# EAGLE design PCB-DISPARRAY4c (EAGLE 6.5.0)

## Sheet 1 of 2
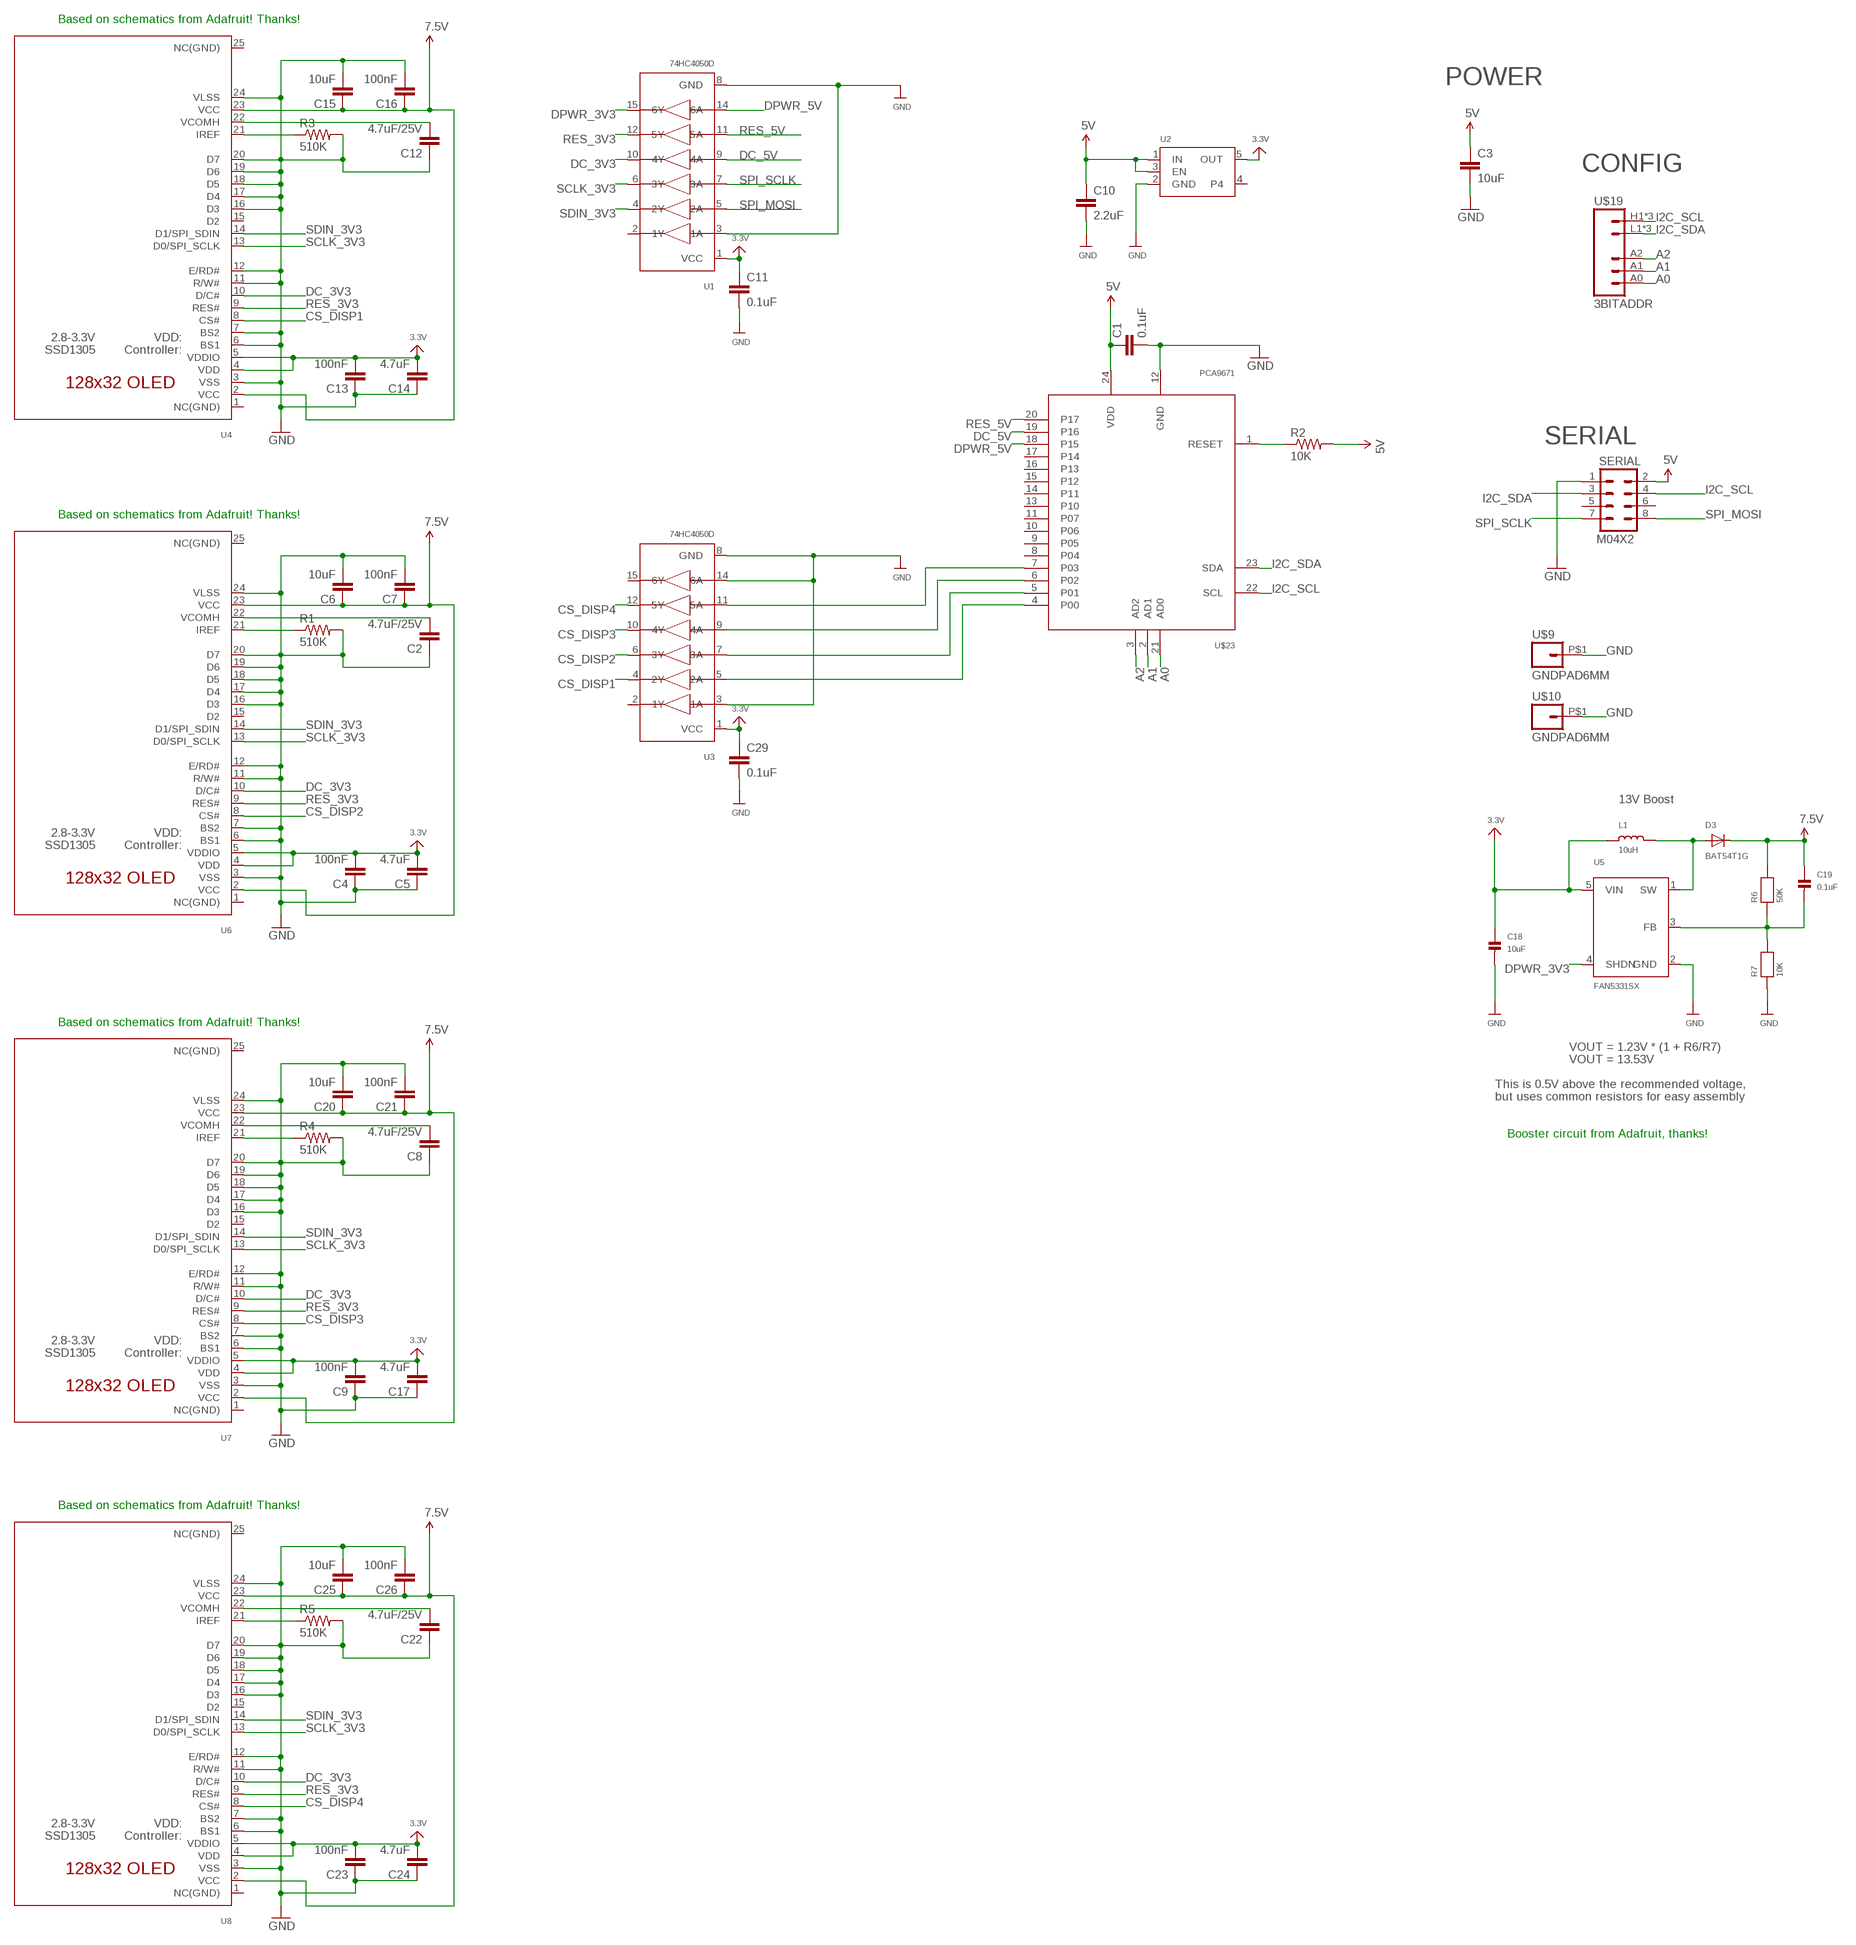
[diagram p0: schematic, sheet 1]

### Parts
C1  0.1uF  CAP0603-CAP  [0603-CAP]
C2  4.7uF/25V  CAP0805  [0805]
C3  10uF  CAP0805  [0805]
C4  100nF  CAP0603-CAP  [0603-CAP]
C5  4.7uF  CAP0603-CAP  [0603-CAP]
C6  10uF  CAP0805  [0805]
C7  100nF  CAP0805  [0805]
C8  4.7uF/25V  CAP0805  [0805]
C9  100nF  CAP0603-CAP  [0603-CAP]
C10  2.2uF  CAP0603-CAP  [0603-CAP]
C11  0.1uF  CAP0603-CAP  [0603-CAP]
C12  4.7uF/25V  CAP0805  [0805]
C13  100nF  CAP0603-CAP  [0603-CAP]
C14  4.7uF  CAP0603-CAP  [0603-CAP]
C15  10uF  CAP0805  [0805]
C16  100nF  CAP0603-CAP  [0603-CAP]
C17  4.7uF  CAP0603-CAP  [0603-CAP]
C18  10uF  CAP_CERAMIC0805  [0805]
C19  0.1uF  CAP_CERAMIC0603  [0603]
C20  10uF  CAP0805  [0805]
C21  100nF  CAP0603-CAP  [0603-CAP]
C22  4.7uF/25V  CAP0805  [0805]
C23  100nF  CAP0603-CAP  [0603-CAP]
C24  4.7uF  CAP0603-CAP  [0603-CAP]
C25  10uF  CAP0805  [0805]
C26  100nF  CAP0603-CAP  [0603-CAP]
C29  0.1uF  CAP0603-CAP  [0603-CAP]
D3  BAT54T1G  DIODESOD-123  [SOD-123]
L1  10uH  INDUCTOR  [INDUCTOR_1007]
R1  510K  RESISTOR0603-RES  [0603-RES]
R2  10K  RESISTOR0603-RES  [0603-RES]
R3  510K  RESISTOR0603-RES  [0603-RES]
R4  510K  RESISTOR0603-RES  [0603-RES]
R5  510K  RESISTOR0603-RES  [0603-RES]
R6  50K  RESISTOR0603  [0603]
R7  10K  RESISTOR0603  [0603]
SERIAL  M04X2  [2X4]
U1  74HC4050D  74HC4050DTSSOP16  [TSSOP16]
U2  VREG_SOT23-5  [SOT23-5]
U3  74HC4050D  74HC4050DTSSOP16  [TSSOP16]
U4  ER-OLED0.91-2TOP  [ER_OLED0.91-2]
U5  FAN5331SX  FAN5331  [SOT23-5]
U6  ER-OLED0.91-2TOP  [ER_OLED0.91-2]
U7  ER-OLED0.91-2TOP  [ER_OLED0.91-2]
U8  ER-OLED0.91-2TOP  [ER_OLED0.91-2]
U$9  GNDPAD6MM  [3.2MMPAD6MM]
U$10  GNDPAD6MM  [3.2MMPAD6MM]
U$19  3BITADDR  [3BITADDR]
U$23  PCA9671  [TSSOP24]

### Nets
3.3V [Power]: C4.2 C5.2 C9.2 C11.1 C13.2 C14.2 C17.2 C18.1 C23.2 C24.2 C29.1 L1.P$1 U1.1(VCC) U2.5(OUT) U3.1(VCC) U4.4(VDD) U4.5(VDDIO) U5.5(VIN) U6.4(VDD) U6.5(VDDIO) U7.4(VDD) U7.5(VDDIO) U8.4(VDD) U8.5(VDDIO)
5V [Power]: C1.1 C3.1 C10.1 R2.2 SERIAL.2 U2.1(IN) U2.3(EN) U$23.24(VDD)
7.5V [Power]: C6.1 C7.1 C15.1 C16.1 C19.1 C20.1 C21.1 C25.1 C26.1 D3.C R6.2 U4.2(VCC) U4.23(VCC) U6.2(VCC) U6.23(VCC) U7.2(VCC) U7.23(VCC) U8.2(VCC) U8.23(VCC)
A0: U$19.A0 U$23.21(AD0)
A1: U$19.A1 U$23.2(AD1)
A2: U$19.A2 U$23.3(AD2)
CS_DISP1: U3.4(2Y) U4.8(CS#)
CS_DISP2: U3.6(3Y) U6.8(CS#)
CS_DISP3: U3.10(4Y) U7.8(CS#)
CS_DISP4: U3.12(5Y) U8.8(CS#)
DC_3V3: U1.10(4Y) U4.10(D/C#) U6.10(D/C#) U7.10(D/C#) U8.10(D/C#)
DC_5V: U1.9(4A) U$23.19(P16)
DPWR_3V3: U1.15(6Y) U5.4(SHDN)
DPWR_5V: U1.14(6A) U$23.18(P15)
GND [Power]: C1.2 C2.1 C3.2 C4.1 C5.1 C6.2 C7.2 C8.1 C9.1 C10.2 C11.2 C12.1 C13.1 C14.1 C15.2 C16.2 C17.1 C18.2 C20.2 C21.2 C22.1 C23.1 C24.1 C25.2 C26.2 C29.2 R1.2 R3.2 R4.2 R5.2 R7.1 SERIAL.1 U1.3(1A) U1.8(GND) U2.2(GND) U3.3(1A) U3.8(GND) U3.14(6A) U4.3(VSS) U4.6(BS1) U4.7(BS2) U4.11(R/W#) U4.12(E/RD#) U4.16(D3) U4.17(D4) U4.18(D5) U4.19(D6) U4.20(D7) U4.24(VLSS) U5.2(GND) U6.3(VSS) U6.6(BS1) U6.7(BS2) U6.11(R/W#) U6.12(E/RD#) U6.16(D3) U6.17(D4) U6.18(D5) U6.19(D6) U6.20(D7) U6.24(VLSS) U7.3(VSS) U7.6(BS1) U7.7(BS2) U7.11(R/W#) U7.12(E/RD#) U7.16(D3) U7.17(D4) U7.18(D5) U7.19(D6) U7.20(D7) U7.24(VLSS) U8.3(VSS) U8.6(BS1) U8.7(BS2) U8.11(R/W#) U8.12(E/RD#) U8.16(D3) U8.17(D4) U8.18(D5) U8.19(D6) U8.20(D7) U8.24(VLSS) U$9.P$1 U$10.P$1 U$23.12(GND)
I2C_SCL: SERIAL.4 U$19.H1(VCC) U$19.H2(VCC) U$19.H3(VCC) U$23.22(SCL)
I2C_SDA: SERIAL.3 U$19.L1(GND) U$19.L2(GND) U$19.L3(GND) U$23.23(SDA)
N$1: R2.1 U$23.1(RESET)
N$2: R1.1 U6.21(IREF)
N$3: C2.2 U6.22(VCOMH)
N$4: R4.1 U7.21(IREF)
N$5: R3.1 U4.21(IREF)
N$6: C8.2 U7.22(VCOMH)
N$7: R5.1 U8.21(IREF)
N$8: C22.2 U8.22(VCOMH)
N$10: C12.2 U4.22(VCOMH)
N$14 [Power]: D3.A L1.P$2 U5.1(SW)
N$15: C19.2 R6.1 R7.2 U5.3(FB)
N$29: U3.5(2A) U$23.4(P00)
N$30: U3.7(3A) U$23.5(P01)
N$31: U3.9(4A) U$23.6(P02)
N$32: U3.11(5A) U$23.7(P03)
RES_3V3: U1.12(5Y) U4.9(RES#) U6.9(RES#) U7.9(RES#) U8.9(RES#)
RES_5V: U1.11(5A) U$23.20(P17)
SCLK_3V3: U1.6(3Y) U4.13(D0/SPI_SCLK) U6.13(D0/SPI_SCLK) U7.13(D0/SPI_SCLK) U8.13(D0/SPI_SCLK)
SDIN_3V3: U1.4(2Y) U4.14(D1/SPI_SDIN) U6.14(D1/SPI_SDIN) U7.14(D1/SPI_SDIN) U8.14(D1/SPI_SDIN)
SPI_MOSI: SERIAL.8 U1.5(2A)
SPI_SCLK: SERIAL.7 U1.7(3A)
Unconnected: SERIAL.5 SERIAL.6 U1.2(1Y) U2.4 U3.2(1Y) U3.15(6Y) U4.1(NC(GND)) U4.15(D2) U4.25(NC(GND)) U6.1(NC(GND)) U6.15(D2) U6.25(NC(GND)) U7.1(NC(GND)) U7.15(D2) U7.25(NC(GND)) U8.1(NC(GND)) U8.15(D2) U8.25(NC(GND)) U$23.8(P04) U$23.9(P05) U$23.10(P06) U$23.11(P07) U$23.13(P10) U$23.14(P11) U$23.15(P12) U$23.16(P13) U$23.17(P14)

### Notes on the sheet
- Based on schematics from Adafruit! Thanks!
- POWER
- CONFIG
- SERIAL
- Based on schematics from Adafruit! Thanks!
- 13V Boost
- Based on schematics from Adafruit! Thanks!
- VOUT = 1.23V * (1 + R6/R7)
- VOUT = 13.53V
- This is 0.5V above the recommended voltage,
- but uses common resistors for easy assembly
- Booster circuit from Adafruit, thanks!
- Based on schematics from Adafruit! Thanks!

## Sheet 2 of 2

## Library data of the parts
C1-C17 C20-C26 C29 = SparkFun:CAP: Capacitor
C18 C19 = microbuilder:CAP_CERAMIC: Ceramic Capacitors
D3 = microbuilder:DIODE: Diode
L1 = microbuilder:INDUCTOR: Inductors
R1-R5 = SparkFun:RESISTOR: Resistor
R6 R7 = microbuilder:RESISTOR: Resistors
SERIAL = SparkFun:M04X2
U1 U3 = SKAARHOJ:74HC4050D: 6-channel level shifter 74HC4050D - 2V-6V Supply Digikey: 74HC4050D,653-ND Mouser: 771-74HC4050D-T
U2 = microbuilder:VREG_SOT23-5: SOT23-5 Fixed Voltage Regulators To better organise some of the SOT23-5 fixed voltage regulators in this library, this new part was created. Part Current Out V Out V In V Dropout Digikey Part No. ADP121 150mA 3.3V 3.4-5.5V 0.09V @ 150mA ADP121-AUJZ33R7CT-ND ADP121 150mA 3.0V 3.1-5.5V 0.09V @ 150mA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
U4 U6-U8 = SKAARHOJ:ER-OLED0.91-2: UG-2864HSWEG01 OLED display Both 1.3" and 0.96" models share the same FPC tab footprint, only the screen dimensions vary.
U5 = microbuilder:FAN5331: FAN5331 - LED/OLED 20V Boost Converter Digikey: FAN5331SXCT-ND
U$9 U$10 = SKAARHOJ:GNDPAD
U$19 = SKAARHOJ:3BITADDR
U$23 = SKAARHOJ:PCA9671

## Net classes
0 default: width 0.203 mm, drill 0.305 mm, clearance 0.152 mm
1 Power: width 0.305 mm, drill 0.406 mm, clearance 0.152 mm

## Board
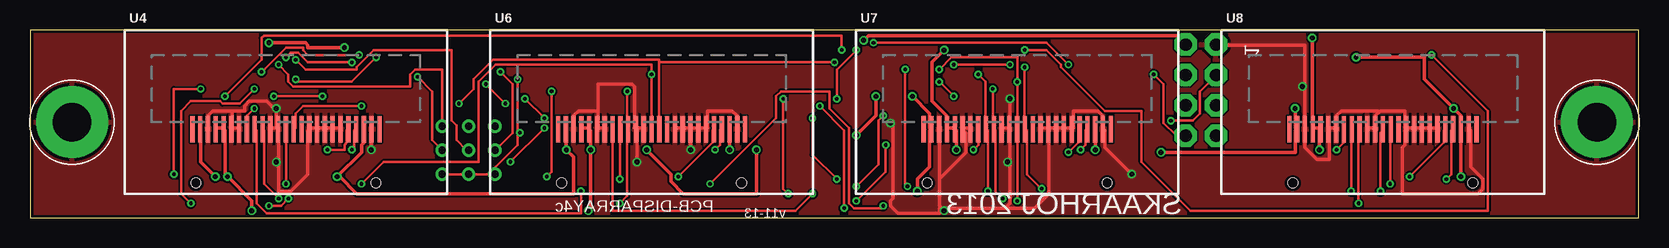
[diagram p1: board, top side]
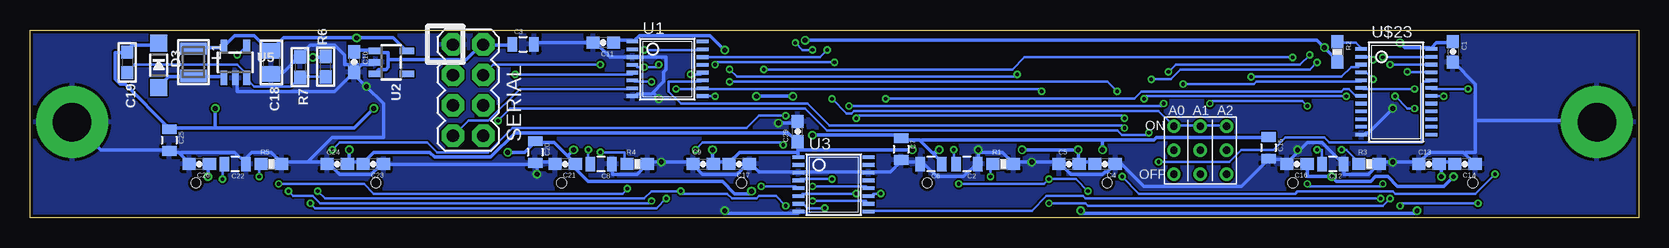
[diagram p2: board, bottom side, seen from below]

Size 134.11 x 15.7 mm. Coordinates in mm from the lower left corner, seen from the top.
Outline: 134.11,0 134.11,15.7 0,15.7 0,0 134.11,0
Copper layers (1*16): Top 0.035mm / dielectric 1.5mm / Bottom 0.035mm
Design rules "Fusion_eagle_rule_v1.1": minimum track width 6mil, minimum drill 12mil, track to track 6mil, track to pad 6mil, pad to pad 6mil, via to via 6mil, smd to smd 0mil, copper to edge 10mil, drill to drill 10mil, minimum pad ring 10mil, minimum via ring 6mil, stop-mask expansion 2mil, vias tented up to drill 100mil, thermal gap 10mil

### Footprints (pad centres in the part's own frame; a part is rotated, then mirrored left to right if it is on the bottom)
0603-CAP = smd 1.1 x 1: 1 -0.85,0; 2 0.85,0
0805 = smd 0.8 x 1.2: 1 -0.9,0; 2 0.9,0
0805' = smd 1.3 x 1.5: 1 -0.95,0; 2 0.95,0
0603 = smd 1.1 x 1: 1 -0.85,0; 2 0.85,0
SOD-123 = smd 1.4 x 1.4: A 1.85,0; C -1.85,0
INDUCTOR_1007 = smd 1.016 x 2.2: P$1 -1.127,0; P$2 1.127,0
0603-RES = smd 1.1 x 1: 1 -0.85,0; 2 0.85,0
2X4 = drill 1.016 pad 1.88 octagon: 1 -3.81,-1.27; 2 -3.81,1.27; 3 -1.27,-1.27; 4 -1.27,1.27; 5 1.27,-1.27; 6 1.27,1.27; 7 3.81,-1.27; 8 3.81,1.27
TSSOP16 = smd 0.305 x 0.991: 1 -3.575,-2.918; 2 -2.925,-2.918; 3 -2.275,-2.918; 4 -1.625,-2.918; 5 -0.975,-2.918; 6 -0.325,-2.918; 7 0.325,-2.918; 8 0.975,-2.918; 9 0.975,2.918; 10 0.325,2.918; 11 -0.325,2.918; 12 -0.975,2.918; 13 -1.625,2.918; 14 -2.275,2.918; 15 -2.925,2.918; 16 -3.575,2.918
SOT23-5 = smd 0.55 x 1.2: 1 -0.95,-1.3; 2 0,-1.3; 3 0.95,-1.3; 4 0.95,1.3; 5 -0.95,1.3
ER_OLED0.91-2 = smd 0.35 x 2.2: 1 -7.8,-1.43; 2 -7.15,-1.43; 3 -6.5,-1.43; 4 -5.85,-1.43; 5 -5.2,-1.43; 6 -4.55,-1.43; 7 -3.9,-1.43; 8 -3.25,-1.43; 9 -2.6,-1.43; 10 -1.95,-1.43; 11 -1.3,-1.43; 12 -0.65,-1.43; 13 0,-1.43; 14 0.65,-1.43; 15 1.3,-1.43; 16 1.95,-1.43; 17 2.6,-1.43; 18 3.25,-1.43; 19 3.9,-1.43; 20 4.55,-1.43; 21 5.2,-1.43; 22 5.85,-1.43; 23 6.5,-1.43; 24 7.15,-1.43; 25 7.8,-1.43 | hole 0.8: -7.5,-5.93; 7.5,-5.93
3.2MMPAD6MM = drill 3.2 pad 6: P$1 0,0
3BITADDR = drill 0.6: A0 -2.2,0; A1 0,0; A2 2.2,0; H1 -2.2,2; H2 0,2; H3 2.2,2; L1 -2.2,-2; L2 0,-2; L3 2.2,-2
TSSOP24 = smd 0.305 x 0.991: 1 -4.225,-2.918; 2 -3.575,-2.918; 3 -2.925,-2.918; 4 -2.275,-2.918; 5 -1.625,-2.918; 6 -0.975,-2.918; 7 -0.325,-2.918; 8 0.325,-2.918; 9 0.975,-2.918; 10 1.625,-2.918; 11 2.275,-2.918; 12 2.925,-2.918; 13 2.925,2.918; 14 2.275,2.918; 15 1.625,2.918; 16 0.975,2.918; 17 0.325,2.918; 18 -0.325,2.918; 19 -0.975,2.918; 20 -1.625,2.918; 21 -2.275,2.918; 22 -2.925,2.918; 23 -3.575,2.918; 24 -4.225,2.918

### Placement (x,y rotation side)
C1  15.49,13.87 270 bottom
C2  56,4.5 180 bottom
C3  93,14.5 0 bottom
C4  44.5,4.5 180 bottom
C5  47.5,4.5 0 bottom
C6  59,4.5 180 bottom
C7  61.5,5.75 270 bottom
C8  86.5,4.5 180 bottom
C9  78,4.5 0 bottom
C10  107.09,13.02 270 bottom
C11  86.32,14.63 180 bottom
C12  25.5,4.5 180 bottom
C13  17.5,4.5 0 bottom
C14  14.5,4.5 180 bottom
C15  30.87,5.87 270 bottom
C16  28.5,4.5 180 bottom
C17  75,4.5 180 bottom
C18  10uF  [0805']  114,13 270 bottom
C19  126,13 270 bottom
C20  92,5.5 270 bottom
C21  89.5,4.5 180 bottom
C22  117,4.5 180 bottom
C23  105.5,4.5 180 bottom
C24  108.5,4.5 0 bottom
C25  122.5,6.5 270 bottom
C26  120,4.5 180 bottom
C29  70.12,7.21 90 bottom
D3  123.37,12.75 270 bottom
L1  120.5,13 270 bottom
R1  53,4.5 0 bottom
R2  25.13,13.88 270 bottom
R3  22.5,4.5 0 bottom
R4  83.5,4.5 0 bottom
R5  114,4.5 0 bottom
R6  109.46,12.64 90 bottom
R7  111.61,12.59 270 bottom
SERIAL  97.6,10.67 270 bottom
U1  80.98,11.16 270 bottom
U2  104,13 270 bottom
U3  67.12,1.51 270 bottom
U4  21.34,8.85 0 top
U5  117,13 0 bottom
U6  51.82,8.85 0 top
U7  82.3,8.85 0 top
U8  112.78,8.85 0 top
U$9  130.61,8 0 top
U$10  3.5,8 0 top
U$19  36.56,5.65 0 bottom
U$23  20.23,9.88 270 bottom

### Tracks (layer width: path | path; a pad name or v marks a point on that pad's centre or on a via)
3.3V  (via drill 0.41)
  Top 0.305: v107.49,5.69 107.49,7.32 U8.5 107.49,7.52 107.09,7.52 U8.4 106.88,7.52 v106.88,15.04 | v76.2,14.02 75.18,13.01 75.18,9.75 76.4,8.53 76.4,7.52 U7.4 76.61,7.52 77.01,7.52 U7.5 77.22,7.32 v77.22,5.69 | U4.4 15.65,7.52 16.05,7.52 U4.5 16.26,7.32 16.26,3.66 v16.46,3.45 18.49,1.42 v18.49,0.61 | U6.4 46.13,7.52 46.53,7.52 U6.5 46.74,7.32 v46.74,5.69 46.74,0.81 v46.53,0.61 | v51.41,5.69 53.44,3.66 53.44,3.05 54.46,2.03 60.55,2.03 v60.55,5.69
  Bottom 0.305: 107.49,4.67 106.48,4.67 C23.2 106.27,4.67 105.46,5.49 100.79,5.49 100.38,5.08 95.71,5.08 93.67,7.11 70.92,7.11 70.31,6.5 C29.1 70.1,6.3 70.1,5.69 | v107.49,5.69 107.49,4.67 | 107.49,4.67 C24.2 | L1.P$1 120.5,14.22 118.06,14.22 U5.5 117.86,14.43 117.04,15.24 115.42,15.24 114.2,14.02 C18.1 114,14.02 112.98,15.04 v106.88,15.04 103.83,15.04 102.82,14.02 U2.5 | C11.1 85.34,14.83 83.92,14.83 U1.1 83.72,14.83 83.31,15.24 77.42,15.24 v76.2,14.02 | C14.2 15.44,4.67 16.46,4.67 C13.2 16.46,4.47 v16.46,3.45 | C4.2 45.52,4.67 46.53,4.67 C5.2 46.74,4.67 v46.74,5.69 v51.41,5.69 | 70.1,5.69 70.1,5.49 | 70.1,5.49 70.1,5.08 U3.1 | 70.1,5.49 74.98,5.49 75.79,4.67 C17.2 76,4.67 77.01,4.67 C9.2 77.22,4.67 v77.22,5.69 | 70.1,5.69 v60.55,5.69 | v18.49,0.61 18.69,0.41 46.33,0.41 v46.53,0.61
5V  (via drill 0.41)
  Top 0.305: v26.21,14.22 23.16,14.22 23.16,14.43 22.96,14.63 v19.91,14.63 | v69.49,14.83 69.9,15.24 96.32,15.24 96.32,14.63 SERIAL.2
  Bottom 0.305: C1.1 15.65,14.63 16.87,14.63 17.27,14.22 U$23.24 17.48,14.22 19.51,14.22 v19.91,14.63 | R2.2 25.2,13.21 v26.21,14.22 26.82,14.83 v69.49,14.83 | C10.1 107.09,14.02 105.46,14.02 U2.1 105.26,13.82 104.24,13.82 104.24,13.21 | 104.24,13.21 104.24,12.6 104.44,12.39 105.05,12.39 105.26,12.19 U2.3 | C3.1 94.08,14.43 96.32,14.43 SERIAL.2 96.52,14.43 97.74,13.21 104.24,13.21
7.5V  (via drill 0.41)
  Top 0.305: v15.44,3.45 14.22,4.67 14.22,7.32 U4.2 | 27.84,7.52 U4.23 27.84,7.32 27.84,6.3 27.64,6.1 27.64,5.49 v25.6,3.45 25.81,3.45 27.23,2.03 45.31,2.03 45.31,5.08 v44.7,5.69 44.7,7.32 U6.2 44.7,7.52 | 58.32,7.52 U6.23 58.32,7.32 v58.32,5.69 | 88.8,7.52 U7.23 88.8,7.32 v88.8,5.69 | 75.18,7.52 U7.2 | v73.97,2.23 73.97,3.25 74.98,4.27 74.98,7.32 U7.2 | v110.54,13.41 116.23,13.41 116.23,11.58 v118.67,9.14 119.28,8.53 119.28,7.52 U8.23 119.28,7.32 v119.28,3.45 | 105.66,7.52 U8.2 | v105.46,9.14 105.46,7.52 U8.2 | v94.28,5.49 105.46,5.49 105.46,7.32 U8.2 | v68.89,6.91 70.51,8.53 v70.51,10.16 | v73.56,10.16 74.98,8.74 74.98,7.52 U7.2
  Bottom 0.305: C16.1 27.64,4.47 27.64,3.45 v25.6,3.45 25.2,3.05 22.35,3.05 21.95,3.45 20.93,3.45 20.12,2.64 16.26,2.64 v15.44,3.45 | 59.84,6.4 59.94,6.5 61.37,6.5 C7.1 61.57,6.71 61.77,6.91 v68.89,6.91 | 59.84,6.4 58.83,5.38 | 58.83,5.38 58.12,4.67 C6.1 | 44.7,6.5 59.74,6.5 59.84,6.4 | 44.7,6.5 40.44,6.5 40.23,6.71 30.89,6.71 C15.1 | 44.7,6.5 v44.7,5.69 | v58.32,5.69 58.52,5.49 58.73,5.49 58.83,5.38 | 89.31,5.18 90.42,6.3 91.85,6.3 C20.1 92.05,6.3 92.86,5.49 v94.28,5.49 | 89.31,5.18 88.8,4.67 C21.1 88.59,4.47 88.59,4.06 87.58,3.05 76.4,3.05 75.39,2.03 74.17,2.03 v73.97,2.23 | 89.31,5.18 v88.8,5.69 | v110.54,13.41 109.53,13.41 R6.2 | v119.28,3.45 119.28,4.47 C26.1 | D3.C 123.55,14.43 125.58,14.43 125.98,14.02 C19.1 126.19,13.82 127,13.82 127,11.58 126.59,11.18 126.19,11.18 122.53,7.52 C25.1 122.33,7.52 118.67,7.52 | v105.46,9.14 107.09,7.52 118.67,7.52 | 118.67,7.52 v118.67,9.14 | v73.56,10.16 v70.51,10.16
A0  (via drill 0.3)
  Top 0.203: v19.3,12.19 21.34,14.22 22.76,14.22 22.76,14.02 23.16,13.61 v27.43,13.61 | v39.22,12.19 40.23,11.18 40.23,7.11 38.81,5.69 U$19.A0
  Bottom 0.203: v19.3,12.19 17.48,12.19 U$23.21 | v27.43,13.61 28.25,12.8 38.61,12.8 v39.22,12.19
A1  (via drill 0.3)
  Top 0.203: v22.15,13.21 22.96,12.39 27.23,12.39 27.23,12.6 28.65,14.02 35.15,14.02 35.15,8.13 35.56,7.72 35.56,6.5 36.37,5.69 U$19.A1
  Bottom 0.203: v22.15,13.21 22.35,13.41 22.96,13.41 U$23.2
A2  (via drill 0.3)
  Top 0.203: v32.31,11.79 33.53,10.57 33.53,6.5 34.34,5.69 U$19.A2
  Bottom 0.203: v32.31,11.79 24.79,11.79 23.98,12.6 23.37,12.6 23.16,12.8 U$23.3
CS_DISP1  (via drill 0.3)
  Top 0.203: v67.26,3.25 65.23,5.28 v65.23,8.33 | v41.25,9.96 v42.88,8.33 | v20.32,10.16 v24.38,10.16 | v18.69,9.14 18.09,8.53 18.09,7.52 U4.8
  Bottom 0.203: v67.26,3.25 69.9,3.25 U3.4 | v65.23,8.33 65.02,8.53 43.08,8.53 v42.88,8.33 | v41.25,9.96 41.05,10.16 v24.38,10.16 | v20.32,10.16 19.3,9.14 v18.69,9.14
CS_DISP2  (via drill 0.3)
  Top 0.203: v65.23,2.03 63.8,0.61 48.56,0.61 48.56,7.32 U6.8
  Bottom 0.203: v65.23,2.03 69.7,2.03 69.9,1.83 U3.6
CS_DISP3  (via drill 0.3)
  Top 0.203: v68.89,1.42 71.32,3.86 v71.32,6.1 | v78.64,5.69 79.05,6.1 79.05,7.32 U7.8
  Bottom 0.203: v68.89,1.42 64.41,1.42 64.21,1.22 U3.10 | v71.32,6.1 71.53,6.3 78.03,6.3 v78.64,5.69
CS_DISP4  (via drill 0.3)
  Top 0.203: v68.89,2.64 70.71,4.47 70.71,8.13 v71.12,8.53 | v108.92,5.69 109.53,6.3 109.53,7.32 U8.8
  Bottom 0.203: v68.89,2.64 64.41,2.64 64.21,2.44 U3.12 | v71.12,8.53 73.36,8.53 74.37,7.52 93.88,7.52 95.91,5.49 100.18,5.49 100.99,6.3 108.31,6.3 v108.92,5.69
DC_3V3  (via drill 0.3)
  Top 0.203: v20.73,1.63 19.51,2.85 19.51,7.32 U4.10 | v49.17,1.22 49.78,1.83 49.78,7.32 U6.10 49.78,7.52 v49.78,10.57 | v80.26,10.77 80.26,7.52 U7.10 80.47,7.32 80.47,2.23 v81.08,1.63 | v110.74,1.22 110.74,7.32 U8.10
  Bottom 0.203: v20.73,1.63 21.34,1.02 45.92,1.02 46.13,1.22 v49.17,1.22 | v80.26,10.77 78.23,10.77 U1.10 78.03,10.77 49.99,10.77 v49.78,10.57 | v110.74,1.22 110.34,0.81 81.89,0.81 v81.08,1.63
DC_5V  (via drill 0.3)
  Top 0.203: v14.22,10.77 11.99,10.77 v11.99,3.66 | v43.08,3.45 43.48,3.86 v43.48,10.57 | v77.01,10.16 v75.79,11.38
  Bottom 0.203: v14.22,10.77 17.27,10.77 U$23.19 | v11.99,3.66 13.61,2.03 20.32,2.03 20.52,2.23 28.45,2.23 28.65,2.03 41.66,2.03 v43.08,3.45 | v43.48,10.57 44.3,11.38 v75.79,11.38 | v77.01,10.16 78.03,10.16 U1.9
DPWR_3V3  (via drill 0.3)
  Top 0.203: v82.91,14.02 84.73,14.02 85.95,12.8 85.95,12.6 89.61,8.94 92.66,8.94 92.66,4.67 96.72,0.61 121.51,0.61 121.51,8.94 v116.84,13.61
  Bottom 0.203: v82.91,14.02 78.23,14.02 U1.15 | v116.84,13.61 116.23,14.22 U5.4
DPWR_5V  (via drill 0.3)
  Top 0.203: v16.26,10.16 19.3,13.21 19.3,15.04 19.51,15.24 67.67,15.24 v67.67,14.02
  Bottom 0.203: v16.26,10.16 17.27,10.16 U$23.18 | v67.67,14.02 68.28,13.41 78.03,13.41 U1.14
GND  (via drill 0.41)
  Top 0.305: U8.20 117.25,7.52 116.84,7.52 U8.19 116.64,7.52 116.03,7.52 | U8.11 111.56,7.52 111.96,7.52 U8.12 112.17,7.52 112.17,8.53 112.47,8.84 | U8.16 114.81,7.52 115.21,7.52 U8.17 115.42,7.52 116.03,7.52 | U8.24 120.09,7.32 120.09,4.27 121.11,3.25 121.11,2.44 120.7,2.03 114.4,2.03 114.4,5.89 114.61,6.1 114.61,7.32 U8.16 | 112.47,8.84 112.57,8.94 114.61,8.94 114.61,7.52 U8.16 | 116.03,7.52 U8.18 | 112.47,8.84 112.37,8.94 109.32,8.94 108.92,8.53 108.92,7.52 U8.7 108.71,7.52 108.31,7.52 U8.6 108.31,7.32 108.31,4.88 107.29,4.88 106.27,5.89 106.27,7.32 U8.3 106.27,7.52 106.27,10.97 | 106.27,10.97 106.27,14.43 98.96,14.43 SERIAL.1 | v106.07,10.97 106.27,10.97 | 16.87,8.94 15.24,8.94 14.83,8.53 14.83,7.52 U4.3 | 16.87,7.52 16.87,8.94 | 16.87,7.52 17.27,7.52 U4.7 | 16.87,7.52 U4.6 | U4.20 25.81,7.52 25.4,7.52 U4.19 25.2,7.52 24.59,7.52 | 24.59,7.52 23.98,7.52 U4.17 23.77,7.52 23.37,7.52 U4.16 23.16,7.32 23.16,3.66 21.74,2.23 20.73,2.23 20.73,4.67 | 24.59,7.52 U4.18 | 20.52,7.52 20.52,8.94 | 20.52,7.52 20.12,7.52 U4.11 | 20.52,7.52 U4.12 20.73,7.32 20.73,4.67 | 16.87,8.94 17.88,8.94 17.88,9.35 18.29,9.75 19.71,9.75 20.52,8.94 | 20.52,8.94 v20.52,9.14 | v28.45,5.69 28.45,7.32 U4.24 | v20.52,4.67 20.73,4.67 | U7.16 84.33,7.52 84.73,7.52 U7.17 | 85.55,7.52 84.94,7.52 U7.17 | 85.55,7.52 86.16,7.52 U7.19 86.36,7.52 86.77,7.52 U7.20 86.97,7.52 86.97,8.94 89,8.94 89.41,8.53 89.41,7.52 U7.24 89.61,7.32 89.61,5.89 v91.85,3.66 | 85.55,7.52 U7.18 | U7.11 81.08,7.52 81.48,7.52 U7.12 | U7.7 78.23,7.52 77.83,7.52 U7.6 77.83,7.32 78.03,7.11 78.03,5.49 75.79,3.25 | 75.89,0.91 75.79,1.02 75.79,3.25
  Top 0.305: 75.89,0.91 v76.2,0.61 76.2,0.81 81.28,0.81 81.38,0.91 | 75.79,3.25 75.79,7.32 U7.3 | v71.73,7.92 71.93,7.72 71.93,1.63 71.73,1.42 71.73,1.02 72.34,0.41 75.79,0.41 75.79,0.81 75.89,0.91 | 81.69,4.67 81.69,1.22 81.38,0.91 | 81.69,4.67 81.69,7.32 U7.12 | U7.17 84.94,7.32 84.94,2.03 83.72,0.81 81.48,0.81 81.38,0.91 | v81.69,9.96 81.69,7.52 U7.12 | U6.11 50.6,7.52 51,7.52 U6.12 | 47.35,8.94 45.72,8.94 45.31,8.53 45.31,7.52 U6.3 | 47.35,7.52 47.35,8.94 | 47.35,7.52 47.75,7.52 U6.7 | 47.35,7.52 U6.6 | 47.35,8.94 47.35,11.18 50.19,11.18 50.39,10.97 50.39,7.52 U6.11 | U6.16 53.85,7.52 54.25,7.52 U6.17 54.46,7.52 55.07,7.52 | U6.24 58.93,7.52 58.93,8.53 58.52,8.94 56.49,8.94 56.49,7.52 U6.20 56.29,7.52 55.88,7.52 U6.19 55.68,7.52 55.07,7.52 | 55.07,7.52 U6.18 55.07,7.32 v55.07,5.69 | v50.6,4.67 50.6,7.32 U6.11 | v81.48,4.67 81.69,4.67
  Bottom 0.305: C18.2 114,12.19 112.98,12.19 111.76,13.41 R7.1 111.56,13.61 110.74,14.43 108.71,14.43 107.9,13.61 107.9,12.8 106.68,12.8 106.58,12.7 | 106.58,12.7 106.48,12.8 105.46,12.8 U2.2 | 106.58,12.7 107.09,12.19 C10.2 | U5.2 116.84,11.58 116.84,10.57 108.71,10.57 107.29,11.99 C10.2 | 121.61,5.38 121.72,5.49 122.33,5.49 C25.2 122.53,5.69 128.22,5.69 130.45,7.92 U$9.P$1 | 121.61,5.38 120.9,4.67 C26.2 | 121.61,5.38 121.51,5.49 117.04,5.49 116.23,4.67 C22.1 116.23,4.88 115.62,5.49 114,5.49 113.18,4.67 R5.2 112.98,4.67 110.95,4.67 | C21.2 90.42,4.67 91.85,4.67 C20.2 | 110.95,4.67 109.53,4.67 C24.1 109.32,4.47 109.12,4.47 108.31,3.66 105.66,3.66 104.85,4.47 C23.1 104.65,4.47 92.05,4.47 C20.2 | 110.95,4.67 108.92,6.71 104.65,6.71 104.65,9.55 v106.07,10.97 107.09,11.99 C10.2 | v20.52,9.14 22.55,7.11 22.76,7.11 22.96,6.91 U$23.12 | 14.53,5.38 14.63,5.49 17.48,5.49 18.29,4.67 C13.1 18.49,4.67 v20.52,4.67 21.54,4.67 R3.2 21.74,4.47 22.55,3.66 24.59,3.66 24.59,4.47 C12.1 24.79,4.67 26.42,6.3 27.64,6.3 28.35,5.59 | 14.53,5.38 13.82,4.67 C14.1 | 13.61,8.13 13.61,5.49 14.43,5.49 14.53,5.38 | 13.61,8.13 13.61,11.18 15.44,13.01 C1.2 | 28.35,5.59 29.26,4.67 C16.2 29.46,4.67 29.67,4.88 30.68,4.88 C15.2 30.89,4.88 33.12,2.64 41.25,2.64 43.08,4.47 43.48,4.47 C4.1 43.69,4.47 44.3,3.86 44.5,3.86 44.7,3.66 47.35,3.66 48.16,4.47 C5.1 48.36,4.67 v50.6,4.67 52.02,4.67 R1.2 52.22,4.67 53.03,5.49 55.07,5.49 | v28.45,5.69 28.35,5.59 | 13.61,8.13 3.66,8.13 U$10.P$1 | 82.19,10.46 81.28,11.38 81.28,12.19 81.08,12.39 81.08,13.41 83.72,13.41 U1.3 83.92,13.41 85.75,13.41 86.97,14.63 C11.2 92.05,14.63 C3.2
  Bottom 0.305: 82.19,10.46 82.3,10.36 83.52,10.36 83.72,10.16 U1.8 | v76.2,0.61 76,0.41 70.1,0.41 U3.8 | v71.73,7.92 70.31,7.92 C29.2 | v81.69,9.96 82.19,10.46 | 55.07,5.49 55.07,4.67 C2.1 55.27,4.47 56.29,3.45 58.52,3.45 59.54,4.47 59.74,4.47 C6.2 59.94,4.67 61.37,4.67 C7.2 61.57,4.67 62.38,3.86 64.01,3.86 U3.14 64.21,3.86 69.9,3.86 U3.3 70.1,3.86 73.36,3.86 73.97,4.47 C17.1 74.17,4.47 74.37,4.47 75.18,3.66 78.03,3.66 78.84,4.47 C9.1 79.05,4.67 v81.48,4.67 82.5,4.67 R4.2 82.7,4.47 83.52,3.66 85.55,3.66 85.55,4.47 C8.1 | 55.07,5.49 v55.07,5.69 | v91.85,3.66 91.85,4.47 C20.2
  pour Top: 0,0 134,0 134,16 0,16
  pour Bottom: 0,0 134,0 134,16 0,16
I2C_SCL  (via drill 0.3)
  Top 0.203: v20.73,12.8 21.54,11.99 21.54,11.38 21.95,10.97 31.7,10.97 31.7,11.99 32.11,12.39 34.34,12.39 34.34,7.72 U$19.H3 | v86.56,12.8 84.73,14.63 v70.31,14.63 | v68.89,14.02 67.26,12.39 v67.26,9.96
  Bottom 0.203: v20.73,12.8 17.48,12.8 U$23.22 | U$19.H3 34.54,7.72 36.37,7.72 U$19.H2 36.58,7.72 38.61,7.72 U$19.H1 38.81,7.72 40.03,8.94 65.43,8.94 65.63,8.74 66.04,8.74 v67.26,9.96 | v86.56,12.8 95.5,12.8 96.32,11.99 SERIAL.4 | v70.31,14.63 69.7,14.02 v68.89,14.02
I2C_SDA  (via drill 0.3)
  Top 0.203: U$19.L3 34.54,3.66 36.37,3.66 U$19.L2 36.58,3.66 38.61,3.66 U$19.L1 38.81,3.66 38.81,4.27 40.64,6.1 40.64,7.11 | v21.34,13.41 21.74,13.82 22.35,13.82 23.16,13.01 v26.82,13.01 | 40.64,7.11 v40.64,11.58 | v95.1,8.13 96.93,8.13 97.54,8.74 97.54,10.57 98.75,11.79 SERIAL.3 | 40.64,7.11 v40.84,7.11
  Bottom 0.203: v21.34,13.41 17.48,13.41 U$23.23 | v26.82,13.01 27.43,12.39 38.2,12.39 39.01,11.58 v40.64,11.58 | v95.1,8.13 94.08,9.14 69.49,9.14 67.67,7.32 43.48,7.32 43.08,6.91 41.05,6.91 v40.84,7.11
N$1
  Bottom 0.203: U$23.1 23.16,14.22 23.57,14.63 24.99,14.63 R2.1
N$2  (via drill 0.3)
  Top 0.203: v54.05,3.45 56.9,6.3 56.9,7.32 U6.21
  Bottom 0.203: v54.05,3.45 54.05,4.47 R1.1
N$3  (via drill 0.3)
  Top 0.203: v57.1,5.69 57.51,6.1 57.51,7.32 U6.22
  Bottom 0.203: v57.1,5.69 57.1,4.67 C2.2
N$4  (via drill 0.3)
  Top 0.203: v86.56,5.49 87.38,6.3 87.38,7.32 U7.21
  Bottom 0.203: v86.56,5.49 84.53,5.49 84.53,4.67 R4.1
N$5  (via drill 0.3)
  Top 0.203: v24.79,5.69 26.21,5.69 26.21,6.1 26.42,6.3 26.42,7.32 U4.21
  Bottom 0.203: v24.79,5.69 24.38,5.69 23.37,4.67 R3.1
N$6  (via drill 0.3)
  Top 0.203: v87.58,5.69 87.99,6.1 87.99,7.32 U7.22
  Bottom 0.203: v87.58,5.69 87.58,4.67 C8.2
N$7  (via drill 0.3)
  Top 0.203: v115.01,3.45 117.86,6.3 117.86,7.32 U8.21
  Bottom 0.203: v115.01,3.45 115.01,4.47 R5.1
N$8  (via drill 0.3)
  Top 0.203: v118.06,3.25 118.47,3.66 118.47,7.32 U8.22
  Bottom 0.203: v118.06,3.25 118.06,4.47 C22.2
N$10  (via drill 0.3)
  Top 0.203: v26.82,5.69 27.03,5.89 27.03,7.32 U4.22
  Bottom 0.203: v26.82,5.69 26.42,5.69 26.42,4.67 C12.2
N$14
  Bottom 0.305: U5.1 118.06,11.79 120.5,11.79 L1.P$2 120.7,11.79 122.53,11.79 123.34,10.97 D3.A
N$15
  Bottom 0.203: R6.1 109.53,11.79 111.56,11.79 R7.2 111.76,11.58 112.37,10.97 115.42,10.97 116.03,11.58 U5.3 116.23,11.79 116.23,12.19 116.84,12.8 125.37,12.8 125.98,12.19 C19.2
N$29  (via drill 0.3)
  Top 0.203: v73.15,2.64 72.95,2.85 v72.95,12.39 | v28.85,13.41 26.82,11.38 22.15,11.38 v22.15,11.58
  Bottom 0.203: v73.15,2.64 70.31,2.64 70.1,2.44 U3.5 | v72.95,12.39 52.22,12.39 51.21,13.41 v28.85,13.41 | v22.15,11.58 22.76,12.19 22.96,12.19 U$23.4
N$30  (via drill 0.3)
  Top 0.203: v39.62,9.55 v38,11.18 | v65.84,9.35 67.87,7.32 v67.87,0.81
  Bottom 0.203: v38,11.18 32.11,11.18 31.9,11.38 23.16,11.38 U$23.5 | v39.62,9.55 39.83,9.35 v65.84,9.35 | v67.87,0.81 69.29,0.81 69.7,1.22 69.9,1.22 U3.7
N$31  (via drill 0.3)
  Top 0.203: v21.54,1.63 20.93,1.02 v19.91,1.02 | v13.41,1.22 12.6,2.03 12.6,8.94 13.41,9.75 15.85,9.75 16.05,9.55 17.48,9.55 v18.69,10.77
  Bottom 0.203: v21.54,1.63 46.13,1.63 46.33,1.83 49.38,1.83 50.6,0.61 64.01,0.61 U3.9 | v19.91,1.02 19.71,1.22 v13.41,1.22 | v18.69,10.77 22.96,10.77 U$23.6
N$32  (via drill 0.3)
  Top 0.203: v63.2,2.03 62.79,2.44 v62.79,9.96
  Bottom 0.203: v63.2,2.03 63.8,2.03 64.01,1.83 U3.11 | v62.79,9.96 42.06,9.96 41.45,10.57 24.79,10.57 24.59,10.77 24.18,10.77 23.57,10.16 23.16,10.16 U$23.7
RES_3V3  (via drill 0.3)
  Top 0.203: v45.92,2.23 45.92,0.41 19.71,0.41 18.9,1.22 18.9,7.32 U4.9 | v49.17,3.25 49.17,7.32 U6.9 | v79.05,11.99 79.65,11.38 79.65,7.52 U7.9 79.86,7.32 v79.86,2.23 | v110.13,2.23 110.13,7.32 U8.9 | v56.69,2.85 62.18,8.33 62.18,10.16 62.59,10.57 66.65,10.57 66.65,9.14 68.28,7.52 68.28,1.22 68.68,0.81 71.12,0.81 v71.12,1.02
  Bottom 0.203: v45.92,2.23 46.94,3.25 v49.17,3.25 49.58,2.85 v56.69,2.85 | v79.05,11.99 78.23,11.99 U1.12 | v110.13,2.23 109.53,1.63 82.91,1.63 82.3,2.23 v79.86,2.23 79.65,2.03 76,2.03 75.59,1.63 73.56,1.63 73.36,1.83 71.93,1.83 v71.12,1.02
RES_5V  (via drill 0.3)
  Top 0.203: v42.88,7.52 v40.03,4.67
  Bottom 0.203: v40.03,4.67 34.14,4.67 33.12,5.69 30.48,5.69 29.46,6.71 26.21,6.71 25.81,6.3 18.09,6.3 18.09,11.18 17.88,11.38 17.48,11.38 U$23.20 | v42.88,7.52 43.08,7.72 67.46,7.72 69.29,9.55 79.86,9.55 80.87,10.57 80.87,11.38 78.23,11.38 U1.11
SCLK_3V3  (via drill 0.3)
  Top 0.203: v21.34,2.85 U4.13 | v27.64,2.85 29.46,4.67 37.39,4.67 37.39,11.38 38.81,12.8 51.82,12.8 v51.82,11.99 U6.13 | v112.57,2.23 112.57,7.11 112.78,7.32 U8.13 | v82.3,1.42 U7.13 v82.3,11.38 82.3,13.41 76.81,13.41 v75.79,12.39
  Bottom 0.203: v21.34,2.85 21.54,2.64 27.43,2.64 v27.64,2.85 | v82.3,11.38 83.72,11.38 U1.6 | v112.57,2.23 112.17,1.83 110.54,1.83 109.93,1.22 82.5,1.22 v82.3,1.42 | v51.82,11.99 52.02,11.79 75.18,11.79 v75.79,12.39
SDIN_3V3  (via drill 0.3)
  Top 0.203: v27.64,9.35 22.76,9.35 22.15,8.74 22.15,7.52 U4.14 | v35.76,9.55 36.98,10.77 36.98,11.58 38.61,13.21 52.43,13.21 52.43,13.01 | 52.43,13.01 52.43,7.52 U6.14 | v82.91,12.6 82.91,7.52 U7.14 83.11,7.32 83.11,3.66 v84.33,2.44 | v113.39,2.85 113.39,7.32 U8.14 | v67.06,13.01 52.43,13.01 | v81.69,12.8 v77.01,12.8
  Bottom 0.203: v27.64,9.35 28.04,9.75 35.56,9.75 v35.76,9.55 | U1.4 83.72,12.8 83.52,12.6 v82.91,12.6 81.89,12.6 v81.69,12.8 | v113.39,2.85 106.27,2.85 105.46,2.03 84.73,2.03 v84.33,2.44 | v67.06,13.01 76.81,13.01 v77.01,12.8
SPI_MOSI  (via drill 0.3)
  Top 0.203: v93.67,11.99 94.49,11.18 94.49,7.92 95.5,6.91 96.32,6.91 SERIAL.8
  Bottom 0.203: v93.67,11.99 83.92,11.99 U1.5
SPI_SCLK
  Bottom 0.203: U1.7 83.92,10.77 93.27,10.77 95.91,8.13 97.54,8.13 98.75,6.91 SERIAL.7

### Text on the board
_tsilk: 1 | PCB-DISPARRAY4c | v11-13 | SKAARHOJ 2013

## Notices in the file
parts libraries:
SparkFun: Licensing: CC v3.0 Share-Alike You are welcome to use this library for commercial purposes.
